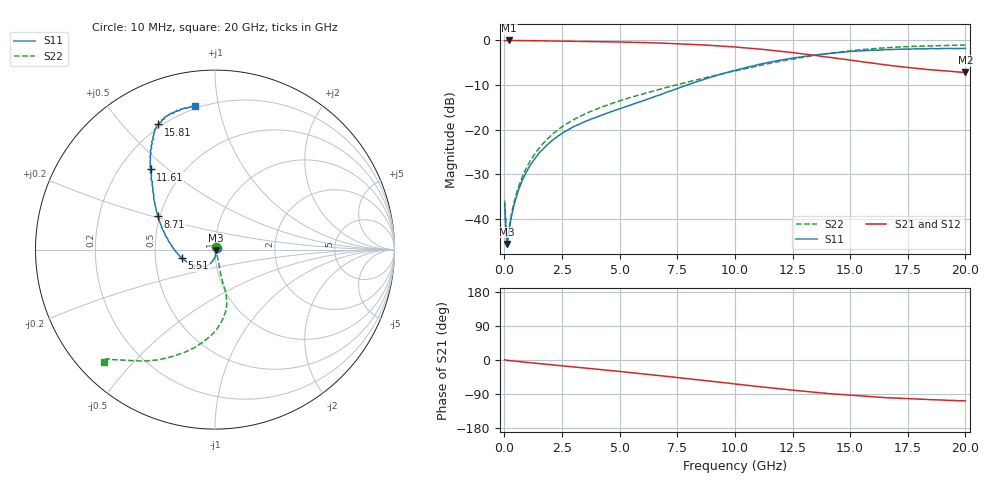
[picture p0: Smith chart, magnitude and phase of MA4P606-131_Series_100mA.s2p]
! AWR Design Environment (9226) Thu Aug 19 15:24:37 2021
! Document = '100mA'
! nPorts: 2, nXvals: 201
# GHz S DB R 50
!Freq DBS11 AngS11 DBS21 AngS21 DBS12 AngS12 DBS22 AngS22
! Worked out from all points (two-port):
!   201 points, 10 MHz to 20 GHz, reference 50 ohm
!   highest |S21| = -0.09 dB at 210 MHz (marker M1); lowest = -7.2 dB at 20 GHz (marker M2)
!   |S21| within 3 dB of the highest: start of sweep to 12.97 GHz
!   lowest |S11| = -45.5 dB at 110 MHz (marker M3), VSWR 1.01, Z = 50.4 - j0.293 ohm
!   |S11| at or under -10 dB: start of sweep to 7.955 GHz
!   |S22| runs from -46.0 to -1.1 dB; largest |S21 - S12| = 0.028
!   S11 on the Smith chart (normalised r, x): 10 MHz: 1.03, +0.02; 5.51 GHz: 0.69, -0.07; 8.71 GHz: 0.49, +0.21; 11.61 GHz: 0.33, +0.44; 15.81 GHz: 0.19, +0.63; 20 GHz: 0.19, +0.85
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0.01  -36.55 29.7  -0.16 0.7  -0.13 0.7  -35.86 59.5
0.11  -45.53 -33.3  -0.09 -0.8  -0.08 -0.7  -46.00 -34.5
0.21  -42.12 -53.0  -0.09 -1.4  -0.08 -1.4  -41.92 -49.1
0.31  -39.38 -63.4  -0.10 -2.1  -0.08 -2.0  -38.75 -58.3
0.41  -36.96 -69.5  -0.10 -2.7  -0.09 -2.7  -36.41 -63.6
0.61  -33.49 -77.8  -0.11 -4.0  -0.10 -3.9  -32.81 -68.2
0.91  -29.88 -85.7  -0.13 -5.9  -0.12 -5.7  -29.02 -70.9
1.21  -27.28 -91.6  -0.15 -7.7  -0.13 -7.5  -26.25 -72.6
1.61  -24.68 -98.5  -0.18 -10.1  -0.16 -9.8  -23.48 -73.8
2.11  -22.26 -106.7  -0.21 -13.0  -0.20 -12.7  -20.91 -75.2
2.61  -20.46 -115.1  -0.25 -16.0  -0.24 -15.6  -18.96 -76.2
3.41  -18.39 -128.5  -0.31 -20.7  -0.29 -20.2  -16.71 -76.8
5.51  -14.45 -165.3  -0.50 -33.4  -0.49 -32.6  -12.75 -76.0
6.71  -12.30 175.0  -0.66 -41.0  -0.64 -40.1  -11.04 -76.8
8.71  -8.71 149.8  -1.12 -54.3  -1.09 -53.0  -8.43 -82.7
10.01  -6.78 138.2  -1.55 -63.3  -1.50 -61.7  -6.91 -89.7
11.61  -4.84 128.8  -2.30 -74.0  -2.19 -72.4  -5.10 -101.6
13.41  -3.39 121.7  -3.38 -84.7  -3.23 -83.6  -3.46 -115.2
15.81  -2.31 114.5  -5.04 -96.5  -4.94 -95.6  -2.01 -129.0
16.71  -2.15 111.5  -5.65 -99.8  -5.61 -98.9  -1.67 -131.9
19.01  -1.88 103.9  -6.83 -105.6  -6.98 -105.2  -1.24 -135.1
20  -1.86 97.9  -7.19 -108.1  -7.42 -107.0  -1.12 -134.8
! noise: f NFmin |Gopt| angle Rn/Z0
0.01  0  1  0  2e-20
2.21  0  1  0  2e-20
4.41  0  1  0  2e-20
6.61  0  1  0  2e-20
8.81  0  1  0  2e-20
11.11  0  1  0  2e-20
13.31  0  1  0  2e-20
15.51  0  1  0  2e-20
17.71  0  1  0  2e-20
20  0  1  0  2e-20
